| z42n_1p1v_it.ibs  *  IBIS 5.0 Model
| 16Gb Mobile LPDDR4 SDRAM - Die Revision E
| This Model is valid for Automotive A2 Temperature Range  -40C<=Ta<=105C
| Part Number   VDD2/VDDQ   Architecture  Package
| SCE11U64324EF   1.10/1.10   1024M x 32   TFBGA (200b,DDP,10x14.5x1.1)
[IBIS Ver]  5.0
[File Name] z42n_0p6v_it.ibs
[Date]   03/31/2025
[File Rev]  2.3
[Source]   Unisemicon, Inc.
[Notes]
   Date   Revision   Contents
   March 31, 2025   1.00   Initial release
[Disclaimer]THESE IBIS MODELS ARE PROVIDED "AS IS" WITH NO WARRANTY AND Unisemicon IS NOT RESPONSIBLE FOR ANY PROBLEMS
   THIS MODEL MAY CAUSE TO THE CUSTOMERS. THESE MODELS ARE SUBJECT TO CHANGE WITHOUT ANY NOTICE.
[Copyright]   Copyright 2025 UniIC, Inc. All rights reserved.
| C_COMP Data:
|   typ   min   max
| DQ   0.834pF   0.784pF   0.884pF
| DQS   0.849pF   0.799pF   0.899pF
| CA_INPUT   0.679pF   0.629pF   0.729pF
| CS_INPUT   0.655pF   0.605pF   0.705pF
| CLK_INPUT   0.656pF   0.606pF   0.706pF
| CKE_INPUT   0.683pF   0.633pF   0.733pF
| ODTCA_INPUT   0.625pF   0.575pF   0.675pF
|COMPONENT:[ SCE11U64324EF ]
[Component]   SCE11U64324EF
[Package Model]  Z42N_200B_SDP_LB2
[Manufacturer]   xxx Technology, Inc.
[Package]
|   typ   min   max
R_pkg   603.13m   431.42m   899.94m
L_pkg   1.668nH   1.132nH   2.472nH
C_pkg   0.609pF   0.467pF   0.865pF
[Pin] signal_name  model_name   R_pin   L_pin   C_pin   | TD_pin(ps)   Z_pin
A1   DNU   NC
A2   DNU   NC
A3   VSS   GND
A4   VDD2   POWER
A5   ZQ   NC
A8   NC   NC
A9   VDD2   POWER
A10   VSS   GND
A11   DNU   NC
A12   DNU   NC
B1   DNU   NC
B2   DQ0   DQ   579.30m   1.530nH   0.601pF   |  30.324   50.455
B3   VDDQ   POWER
B4   DQ7   DQ   521.60m   1.376nH   0.535pF   |  27.132   50.715
B5   VDDQ   POWER
B8   VDDQ   POWER
B9   DQ15   DQ   521.58m   1.381nH   0.535pF   |  27.182   50.807
B10   VDDQ   POWER
B11   DQ8   DQ   582.09m   1.533nH   0.605pF   |  30.454   50.338
B12   DNU   NC
C1   VSS   GND
C2   DQ1   DQ   508.10m   1.311nH   0.554pF   |  26.950   48.646
C3   DMI0   DQ   443.13m   1.164nH   0.502pF   |  24.173   48.153
C4   DQ6   DQ   454.87m   1.195nH   0.489pF   |  24.173   49.434
C5   VSS   GND
C8   VSS   GND
C9   DQ14   DQ   452.17m   1.190nH   0.488pF   |  24.098   49.381
C10   DMI1   DQ   446.55m   1.178nH   0.502pF   |  24.318   48.442
C11   DQ9   DQ   508.55m   1.324nH   0.556pF   |  27.132   48.799
C12   VSS   GND
D1   VDDQ   POWER
D2   VSS   GND
D3   DQS0_t   DQS   651.43m   1.905nH   0.628pF   |  34.588   55.077
D4   VSS   GND
D5   VDDQ   POWER
D8   VDDQ   POWER
D9   VSS   GND
D10   DQS1_t   DQS   651.42m   1.914nH   0.629pF   |  34.697   55.163
D11   VSS   GND
D12   VDDQ   POWER
E1   VSS   GND
E2   DQ2   DQ   500.68m   1.348nH   0.529pF   |  26.704   50.480
E3   DQS0_c   DQS   643.34m   1.890nH   0.601pF   |  33.703   56.078
E4   DQ5   DQ   431.42m   1.168nH   0.481pF   |  23.702   49.278
E5   VSS   GND
E8   VSS   GND
E9   DQ13   DQ   431.43m   1.169nH   0.486pF   |  23.836   49.044
E10   DQS1_c   DQS   643.50m   1.890nH   0.601pF   |  33.703   56.078
E11   DQ10   DQ   500.70m   1.345nH   0.529pF   |  26.674   50.424
E12   VSS   GND
F1   VDD1   POWER
F2   DQ3   DQ   550.84m   1.447nH   0.577pF   |  28.895   50.078
F3   VDDQ   POWER
F4   DQ4   DQ   438.89m   1.132nH   0.467pF   |  22.992   49.234
F5   VDD2   POWER
F8   VDD2   POWER
F9   DQ12   DQ   438.92m   1.132nH   0.472pF   |  23.115   48.972
F10   VDDQ   POWER
F11   DQ11   DQ   550.98m   1.456nH   0.577pF   |  28.985   50.233
F12   VDD1   POWER
G1   VSS   GND
G2   ODT_CA   ODTCA_INPUT   748.07m   2.139nH   0.691pF   |  38.445   55.637
G3   VSS   GND
G4   VDD1   POWER
G5   VSS   GND
G8   VSS   GND
G9   VDD1   POWER
G10   VSS   GND
G11   NC   NC
G12   VSS   GND
H1   VDD2   POWER
H2   CA0   CA_INPUT   811.90m   2.235nH   0.759pF   |  41.187   54.265
H3   NC   NC
H4   CS   CS_INPUT   646.92m   1.910nH   0.647pF   |  35.154   54.333
H5   VDD2   POWER
H8   VDD2   POWER
H9   CA2   CA_INPUT   693.42m   1.911nH   0.688pF   |  36.260   52.703
H10   CA3   CA_INPUT   772.58m   2.175nH   0.746pF   |  40.281   53.996
H11   CA4   CA_INPUT   845.75m   2.405nH   0.802pF   |  43.918   54.761
H12   VDD2   POWER
J1   VSS   GND
J2   CA1   CA_INPUT   872.08m   2.359nH   0.844pF   |  44.621   52.868
J3   VSS   GND
J4   CKE   CKE_INPUT   683.83m   2.042nH   0.679pF   |  37.236   54.839
J5   NC   NC
J8   CK_t   CLK_INPUT   739.69m   2.222nH   0.719pF   |  39.970   55.591
J9   CK_c   CLK_INPUT   737.69m   2.200nH   0.716pF   |  39.689   55.431
J10   VSS   GND
J11   CA5   CA_INPUT   899.94m   2.472nH   0.865pF   |  46.242   53.458
J12   VSS   GND
K1   VDD2   POWER
K2   VSS   GND
K3   VDD2   POWER
K4   VSS   GND
K5   NC   NC
K8   NC   NC
K9   VSS   GND
K10   VDD2   POWER
K11   VSS   GND
K12   VDD2   POWER
N1   VDD2   POWER
N2   VSS   GND
N3   VDD2   POWER
N4   VSS   GND
N5   NC   NC
N8   NC   NC
N9   VSS   GND
N10   VDD2   POWER
N11   VSS   GND
N12   VDD2   POWER
P1   VSS   GND
P2   NC   NC
P3   VSS   GND
P4   NC   NC
P5   NC   NC
P8   NC   NC
P9   NC   NC
P10   VSS   GND
P11   NC   NC
P12   VSS   GND
R1   VDD2   POWER
R2   NC   NC
R3   NC   NC
R4   NC   NC
R5   VDD2   POWER
R8   VDD2   POWER
R9   NC   NC
R10   NC   NC
R11   NC   NC
R12   VDD2   POWER
T1   VSS   GND
T2   NC   NC
T3   VSS   GND
T4   VDD1   POWER
T5   VSS   GND
T8   VSS   GND
T9   VDD1   POWER
T10   VSS   GND
T11   RESET_n   NC
T12   VSS   GND
U1   VDD1   POWER
U2   NC   NC
U3   VDDQ   POWER
U4   NC   NC
U5   VDD2   POWER
U8   VDD2   POWER
U9   NC   NC
U10   VDDQ   POWER
U11   NC   NC
U12   VDD1   POWER
V1   VSS   GND
V2   NC   NC
V3   NC   NC
V4   NC   NC
V5   VSS   GND
V8   VSS   GND
V9   NC   NC
V10   NC   NC
V11   NC   NC
V12   VSS   GND
W1   VDDQ   POWER
W2   VSS   GND
W3   NC   NC
W4   VSS   GND
W5   VDDQ   POWER
W8   VDDQ   POWER
W9   VSS   GND
W10   NC   NC
W11   VSS   GND
W12   VDDQ   POWER
Y1   VSS   GND
Y2   NC   NC
Y3   NC   NC
Y4   NC   NC
Y5   VSS   GND
Y8   VSS   GND
Y9   NC   NC
Y10   NC   NC
Y11   NC   NC
Y12   VSS   GND
AA1   DNU   NC
AA2   NC   NC
AA3   VDDQ   POWER
AA4   NC   NC
AA5   VDDQ   POWER
AA8   VDDQ   POWER
AA9   NC   NC
AA10  VDDQ   POWER
AA11  NC   NC
AA12  DNU   NC
AB1   DNU   NC
AB2   DNU   NC
AB3   VSS   GND
AB4   VDD2   POWER
AB5   VSS   GND
AB8   VSS   GND
AB9   VDD2   POWER
AB10  VSS   GND
AB11  DNU   NC
AB12  DNU   NC
|*****  PIN MAPPING  *******************************************************
[Pin Mapping] pulldown_ref pullup_ref gnd_clamp_ref power_clamp_ref ext_ref
A1   NC   NC
A2   NC   NC
A3   VSS   NC
A4   NC   VDD2
A5   NC   NC
A8   NC   NC
A9   NC   VDD2
A10   VSS   NC
A11   NC   NC
A12   NC   NC
B1   NC   NC
B2   VSS   VDDQ   VSS   VDDQ
B3   NC   VDDQ
B4   VSS   VDDQ   VSS   VDDQ
B5   NC   VDDQ
B8   NC   VDDQ
B9   VSS   VDDQ   VSS   VDDQ
B10   NC   VDDQ
B11   VSS   VDDQ   VSS   VDDQ
B12   NC   NC
C1   VSS   NC
C2   VSS   VDDQ   VSS   VDDQ
C3   VSS   VDDQ   VSS   VDDQ
C4   VSS   VDDQ   VSS   VDDQ
C5   VSS   NC
C8   VSS   NC
C9   VSS   VDDQ   VSS   VDDQ
C10   VSS   VDDQ   VSS   VDDQ
C11   VSS   VDDQ   VSS   VDDQ
C12   VSS   NC
D1   NC   VDDQ
D2   VSS   NC
D3   VSS   VDDQ   VSS   VDDQ
D4   VSS   NC
D5   NC   VDDQ
D8   NC   VDDQ
D9   VSS   NC
D10   VSS   VDDQ   VSS   VDDQ
D11   VSS   NC
D12   NC   VDDQ
E1   VSS   NC
E2   VSS   VDDQ   VSS   VDDQ
E3   VSS   VDDQ   VSS   VDDQ
E4   VSS   VDDQ   VSS   VDDQ
E5   VSS   NC
E8   VSS   NC
E9   VSS   VDDQ   VSS   VDDQ
E10   VSS   VDDQ   VSS   VDDQ
E11   VSS   VDDQ   VSS   VDDQ
E12   VSS   NC
F1   NC   VDD1
F2   VSS   VDDQ   VSS   VDDQ
F3   NC   VDDQ
F4   VSS   VDDQ   VSS   VDDQ
F5   NC   VDD2
F8   NC   VDD2
F9   VSS   VDDQ   VSS   VDDQ
F10   NC   VDDQ
F11   VSS   VDDQ   VSS   VDDQ
F12   NC   VDD1
G1   VSS   NC
G2   NC   NC   VSS   VDD2
G3   VSS   NC
G4   NC   VDD1
G5   VSS   NC
G8   VSS   NC
G9   NC   VDD1
G10   VSS   NC
G11   NC   NC
G12   VSS   NC
H1   NC   VDD2
H2   NC   NC   VSS   VDD2
H3   NC   NC
H4   NC   NC   VSS   VDD2
H5   NC   VDD2
H8   NC   VDD2
H9   NC   NC   VSS   VDD2
H10   NC   NC   VSS   VDD2
H11   NC   NC   VSS   VDD2
H12   NC   VDD2
J1   VSS   NC
J2   NC   NC   VSS   VDD2
J3   VSS   NC
J4   NC   NC   VSS   VDD2
J5   NC   NC
J8   NC   NC   VSS   VDD2
J9   NC   NC   VSS   VDD2
J10   VSS   NC
J11   NC   NC   VSS   VDD2
J12   VSS   NC
K1   NC   VDD2
K2   VSS   NC
K3   NC   VDD2
K4   VSS   NC
K5   NC   NC
K8   NC   NC
K9   VSS   NC
K10   NC   VDD2
K11   VSS   NC
K12   NC   VDD2
N1   NC   VDD2
N2   VSS   NC
N3   NC   VDD2
N4   VSS   NC
N5   NC   NC
N8   NC   NC
N9   VSS   NC
N10   NC   VDD2
N11   VSS   NC
N12   NC   VDD2
P1   VSS   NC
P2   NC   NC
P3   VSS   NC
P4   NC   NC
P5   NC   NC
P8   NC   NC
P9   NC   NC
P10   VSS   NC
P11   NC   NC
P12   VSS   NC
R1   NC   VDD2
R2   NC   NC
R3   NC   NC
R4   NC   NC
R5   NC   VDD2
R8   NC   VDD2
R9   NC   NC
R10   NC   NC
R11   NC   NC
R12   NC   VDD2
T1   VSS   NC
T2   NC   NC
T3   VSS   NC
T4   NC   VDD1
T5   VSS   NC
T8   VSS   NC
T9   NC   VDD1
T10   VSS   NC
T11   NC   NC
T12   VSS   NC
U1   NC   VDD1
U2   NC   NC
U3   NC   VDDQ
U4   NC   NC
U5   NC   VDD2
U8   NC   VDD2
U9   NC   NC
U10   NC   VDDQ
U11   NC   NC
U12   NC   VDD1
V1   VSS   NC
V2   NC   NC
V3   NC   NC
V4   NC   NC
V5   VSS   NC
V8   VSS   NC
V9   NC   NC
V10   NC   NC
V11   NC   NC
V12   VSS   NC
W1   NC   VDDQ
W2   VSS   NC
W3   NC   NC
W4   VSS   NC
W5   NC   VDDQ
W8   NC   VDDQ
W9   VSS   NC
W10   NC   NC
W11   VSS   NC
W12   NC   VDDQ
Y1   VSS   NC
Y2   NC   NC
Y3   NC   NC
Y4   NC   NC
Y5   VSS   NC
Y8   VSS   NC
Y9   NC   NC
Y10   NC   NC
Y11   NC   NC
Y12   VSS   NC
AA1   NC   NC
AA2   NC   NC
AA3   NC   VDDQ
AA4   NC   NC
AA5   NC   VDDQ
AA8   NC   VDDQ
AA9   NC   NC
AA10   NC   VDDQ
AA11   NC   NC
AA12   NC   NC
AB1   NC   NC
AB2   NC   NC
AB3   VSS   NC
AB4   NC   VDD2
AB5   VSS   NC
AB8   VSS   NC
AB9   NC   VDD2
AB10   VSS   NC
AB11   NC   NC
AB12   NC   NC
|*****  DIFF PIN  **********************************************************
[Diff Pin]  inv_pin  vdiff   tdelay_typ   tdelay_min   tdelay_max
D3   E3   0.120V   0.000s   NA   NA
D10   E10   0.120V   0.000s   NA   NA
J8   J9   0.145V   0.000s   NA   NA
|END COMPONENT *************************************************************
|COMPONENT:[ MT53E1G32D2FW ]
[Component]   MT53E1G32D2FW
[Package Model]  Z42N_200B_DDP_LB2
[Manufacturer]   xxx Technology, Inc.
[Package]
|   typ   min   max
R_pkg   1781m   683m   3340m
L_pkg   3.313nH   1.222nH   6.06nH
C_pkg   1.15pF   0.604pF   2.03pF
[Pin] signal_name  model_name   R_pin   L_pin   C_pin
A1   DNU   NC
A2   DNU   NC
A3   VSS   GND
A4   VDD2   POWER
A5   ZQ0   NC
A8   ZQ1   NC
A9   VDD2   POWER
A10   VSS   GND
A11   DNU   NC
A12   DNU   NC
B1   DNU   NC
B2   DQ0_A   DQ   892.22m   1.783nH   0.667pF
B3   VDDQ   POWER
B4   DQ7_A   DQ   942.05m   1.831nH   0.712pF
B5   VDDQ   POWER
B8   VDDQ   POWER
B9   DQ15_A   DQ   905.71m   1.724nH   0.652pF
B10   VDDQ   POWER
B11   DQ8_A   DQ   951.2m   1.847nH   0.708pF
B12   DNU   NC
C1   VSS   GND
C2   DQ1_A   DQ   869.4m   1.675nH   0.663pF
C3   DMI0_A   DQ   802.2m   1.539nH   0.644pF
C4   DQ6_A   DQ   695.07m   1.386nH   0.604pF
C5   VSS   GND
C8   VSS   GND
C9   DQ14_A   DQ   809.8m   1.568nH   0.657pF
C10   DMI1_A   DQ   843.49m   1.585nH   0.669pF
C11   DQ9_A   DQ   862.4m   1.663nH   0.667pF
C12   VSS   GND
D1   VDDQ   POWER
D2   VSS   GND
D3   DQS0_t_A   DQS   872.77m   1.603nH   0.663pF
D4   VSS   GND
D5   VDDQ   POWER
D8   VDDQ   POWER
D9   VSS   GND
D10   DQS1_t_A   DQS   906.95m   1.659nH   0.687pF
D11   VSS   GND
D12   VDDQ   POWER
E1   VSS   GND
E2   DQ2_A   DQ   766.79m   1.41nH   0.641pF
E3   DQS0_c_A   DQS   892.7m   1.616nH   0.682pF
E4   DQ5_A   DQ   683.1m   1.243nH   0.617pF
E5   VSS   GND
E8   VSS   GND
E9   DQ13_A   DQ   751.68m   1.328nH   0.636pF
E10   DQS1_c_A   DQS   932m   1.697nH   0.709pF
E11   DQ10_A   DQ   805.68m   1.499nH   0.658pF
E12   VSS   GND
F1   VDD1   POWER
F2   DQ3_A   DQ   815.2m   1.487nH   0.658pF
F3   VDDQ   POWER
F4   DQ4_A   DQ   684.7m   1.222nH   0.624pF
F5   VDD2   POWER
F8   VDD2   POWER
F9   DQ12_A   DQ   754m   1.333nH   0.665pF
F10   VDDQ   POWER
F11   DQ11_A   DQ   816.75m   1.527nH   0.656pF
F12   VDD1   POWER
G1   VSS   GND
G2   ODT_CA_A   ODTCA_INPUT   3223m   5.38nH   0.839pF
G3   VSS   GND
G4   VDD1   POWER
G5   VSS   GND
G8   VSS   GND
G9   VDD1   POWER
G10   VSS   GND
G11   NC   NC
G12   VSS   GND
H1   VDD2   POWER
H2   CA0_A   CA_INPUT   1381m   2.44nH   0.952pF
H3   NC   NC
H4   CS0_A   CS_INPUT
H5   VDD2   POWER
H8   VDD2   POWER
H9   CA2_A   CA_INPUT   1146m   2.055nH   0.856pF
H10   CA3_A   CA_INPUT   1283m   2.28nH   0.92pF
H11   CA4_A   CA_INPUT   1456m   2.59nH   1.005pF
H12   VDD2   POWER
J1   VSS   GND
J2   CA1_A   CA_INPUT   1531m   2.64nH   1.061pF
J3   VSS   GND
J4   CKE0_A   CKE_INPUT
J5   NC   NC
J8   CK_t_A   CLK_INPUT   1327m   2.423nH   0.917pF
J9   CK_c_A   CLK_INPUT   1352m   2.46nH   0.936pF
J10   VSS   GND
J11   CA5_A   CA_INPUT   1682m   2.901nH   1.08pF
J12   VSS   GND
K1   VDD2   POWER
K2   VSS   GND
K3   VDD2   POWER
K4   VSS   GND
K5   NC   NC
K8   NC   NC
K9   VSS   GND
K10   VDD2   POWER
K11   VSS   GND
K12   VDD2   POWER
N1   VDD2   POWER
N2   VSS   GND
N3   VDD2   POWER
N4   VSS   GND
N5   NC   NC
N8   NC   NC
N9   VSS   GND
N10   VDD2   POWER
N11   VSS   GND
N12   VDD2   POWER
P1   VSS   GND
P2   CA1_B   CA_INPUT   2001m   3.59nH   1.24pF
P3   VSS   GND
P4   CKE0_B   CKE_INPUT
P5   NC   NC
P8   CK_t_B   CLK_INPUT   1908m   3.371nH   1.215pF
P9   CK_c_B   CLK_INPUT   1352m   2.464nH   0.936pF
P10   VSS   GND
P11   CA5_B   CA_INPUT   1935m   3.552nH   1.192pF
P12   VSS   GND
R1   VDD2   POWER
R2   CA0_B   CA_INPUT   2110m   3.79nH   1.283pF
R3   NC   NC
R4   CS0_B   CS_INPUT
R5   VDD2   POWER
R8   VDD2   POWER
R9   CA2_B   CA_INPUT   1965m   3.398nH   1.229pF
R10   CA3_B   CA_INPUT   2061m   3.706nH   1.26pF
R11   CA4_B   CA_INPUT   1859m   3.388nH   1.151pF
R12   VDD2   POWER
T1   VSS   GND
T2   ODT_CA_B   ODTCA_INPUT   1974m   3.548nH   1.128pF
T3   VSS   GND
T4   VDD1   POWER
T5   VSS   GND
T8   VSS   GND
T9   VDD1   POWER
T10   VSS   GND
T11   RESET_n   NC
T12   VSS   GND
U1   VDD1   POWER
U2   DQ3_B   DQ   2687m   4.766nH   1.558pF
U3   VDDQ   POWER
U4   DQ4_B   DQ   2425m   4.233nH   1.469pF
U5   VDD2   POWER
U8   VDD2   POWER
U9   DQ12_B   DQ   3116m   5.207nH   1.812pF
U10   VDDQ   POWER
U11   DQ11_B   DQ   3179m   5.321nH   1.828pF
U12   VDD1   POWER
V1   VSS   GND
V2   DQ2_B   DQ   2588m   4.551nH   1.513pF
V3   DQS0_c_B   DQS   2438m   4.346nH   1.466pF
V4   DQ5_B   DQ   2290m   4.012nH   1.391pF
V5   VSS   GND
V8   VSS   GND
V9   DQ13_B   DQ   3013m   5.038nH   1.759pF
V10   DQS1_c_B   DQS   3073m   5.198nH   1.833pF
V11   DQ10_B   DQ   3240m   5.404nH   1.898pF
V12   VSS   GND
W1   VDDQ   POWER
W2   VSS   GND
W3   DQS0_t_B   DQS   2438m   4.346nH   1.466pF
W4   VSS   GND
W5   VDDQ   POWER
W8   VDDQ   POWER
W9   VSS   GND
W10   DQS1_t_B   DQS   3167m   5.386nH   1.871pF
W11   VSS   GND
W12   VDDQ   POWER
Y1   VSS   GND
Y2   DQ1_B   DQ   2484m   4.410nH   1.467pF
Y3   DMI0_B   DQ   2282m   4.056nH   1.378pF
Y4   DQ6_B   DQ   2149m   3.822nH   1.313pF
Y5   VSS   GND
Y8   VSS   GND
Y9   DQ14_B   DQ   3051m   5.183nH   1.804pF
Y10   DMI1_B   DQ   3195m   5.155nH   1.899pF
Y11   DQ9_B   DQ   3347m   5.68nH   1.932pF
Y12   VSS   GND
AA1   DNU   NC
AA2   DQ0_B   DQ   2472m   4.484nH   1.453pF
AA3   VDDQ   POWER
AA4   DQ7_B   DQ   2196m   4.004nH   1.284pF
AA5   VDDQ   POWER
AA8   VDDQ   POWER
AA9   DQ15_B   DQ   3046m   5.081nH   1.82pF
AA10  VDDQ   POWER
AA11  DQ8_B   DQ   3565m   6.06nH   2.037pF
AA12  DNU   NC
AB1   DNU   NC
AB2   DNU   NC
AB3   VSS   GND
AB4   VDD2   POWER
AB5   VSS   GND
AB8   VSS   GND
AB9   VDD2   POWER
AB10  VSS   GND
AB11  DNU   NC
AB12  DNU   NC
|*****  PIN MAPPING  *******************************************************
[Pin Mapping] pulldown_ref pullup_ref gnd_clamp_ref power_clamp_ref ext_ref
A1   NC   NC
A2   NC   NC
A3   VSS   NC
A4   NC   VDD2
A5   NC   NC
A8   NC   NC
A9   NC   VDD2
A10   VSS   NC
A11   NC   NC
A12   NC   NC
B1   NC   NC
B2   VSS   VDDQ   VSS   VDDQ
B3   NC   VDDQ
B4   VSS   VDDQ   VSS   VDDQ
B5   NC   VDDQ
B8   NC   VDDQ
B9   VSS   VDDQ   VSS   VDDQ
B10   NC   VDDQ
B11   VSS   VDDQ   VSS   VDDQ
B12   NC   NC
C1   VSS   NC
C2   VSS   VDDQ   VSS   VDDQ
C3   VSS   VDDQ   VSS   VDDQ
C4   VSS   VDDQ   VSS   VDDQ
C5   VSS   NC
C8   VSS   NC
C9   VSS   VDDQ   VSS   VDDQ
C10   VSS   VDDQ   VSS   VDDQ
C11   VSS   VDDQ   VSS   VDDQ
C12   VSS   NC
D1   NC   VDDQ
D2   VSS   NC
D3   VSS   VDDQ   VSS   VDDQ
D4   VSS   NC
D5   NC   VDDQ
D8   NC   VDDQ
D9   VSS   NC
D10   VSS   VDDQ   VSS   VDDQ
D11   VSS   NC
D12   NC   VDDQ
E1   VSS   NC
E2   VSS   VDDQ   VSS   VDDQ
E3   VSS   VDDQ   VSS   VDDQ
E4   VSS   VDDQ   VSS   VDDQ
E5   VSS   NC
E8   VSS   NC
E9   VSS   VDDQ   VSS   VDDQ
E10   VSS   VDDQ   VSS   VDDQ
E11   VSS   VDDQ   VSS   VDDQ
E12   VSS   NC
F1   NC   VDD1
F2   VSS   VDDQ   VSS   VDDQ
F3   NC   VDDQ
F4   VSS   VDDQ   VSS   VDDQ
F5   NC   VDD2
F8   NC   VDD2
F9   VSS   VDDQ   VSS   VDDQ
F10   NC   VDDQ
F11   VSS   VDDQ   VSS   VDDQ
F12   NC   VDD1
G1   VSS   NC
G2   NC   NC   VSS   VDD2
G3   VSS   NC
G4   NC   VDD1
G5   VSS   NC
G8   VSS   NC
G9   NC   VDD1
G10   VSS   NC
G11   NC   NC
G12   VSS   NC
H1   NC   VDD2
H2   NC   NC   VSS   VDD2
H3   NC   NC
H4   NC   NC   VSS   VDD2
H5   NC   VDD2
H8   NC   VDD2
H9   NC   NC   VSS   VDD2
H10   NC   NC   VSS   VDD2
H11   NC   NC   VSS   VDD2
H12   NC   VDD2
J1   VSS   NC
J2   NC   NC   VSS   VDD2
J3   VSS   NC
J4   NC   NC   VSS   VDD2
J5   NC   NC
J8   NC   NC   VSS   VDD2
J9   NC   NC   VSS   VDD2
J10   VSS   NC
J11   NC   NC   VSS   VDD2
J12   VSS   NC
K1   NC   VDD2
K2   VSS   NC
K3   NC   VDD2
K4   VSS   NC
K5   NC   NC
K8   NC   NC
K9   VSS   NC
K10   NC   VDD2
K11   VSS   NC
K12   NC   VDD2
N1   NC   VDD2
N2   VSS   NC
N3   NC   VDD2
N4   VSS   NC
N5   NC   NC
N8   NC   NC
N9   VSS   NC
N10   NC   VDD2
N11   VSS   NC
N12   NC   VDD2
P1   VSS   NC
P2   NC   NC   VSS   VDD2
P3   VSS   NC
P4   NC   NC   VSS   VDD2
P5   NC   NC
P8   NC   NC   VSS   VDD2
P9   NC   NC   VSS   VDD2
P10   VSS   NC
P11   NC   NC   VSS   VDD2
P12   VSS   NC
R1   NC   VDD2
R2   NC   NC   VSS   VDD2
R3   NC   NC
R4   NC   NC   VSS   VDD2
R5   NC   VDD2
R8   NC   VDD2
R9   NC   NC   VSS   VDD2
R10   NC   NC   VSS   VDD2
R11   NC   NC   VSS   VDD2
R12   NC   VDD2
T1   VSS   NC
T2   NC   NC   VSS   VDD2
T3   VSS   NC
T4   NC   VDD1
T5   VSS   NC
T8   VSS   NC
T9   NC   VDD1
T10   VSS   NC
T11   NC   NC
T12   VSS   NC
U1   NC   VDD1
U2   VSS   VDDQ   VSS   VDDQ
U3   NC   VDDQ
U4   VSS   VDDQ   VSS   VDDQ
U5   NC   VDD2
U8   NC   VDD2
U9   VSS   VDDQ   VSS   VDDQ
U10   NC   VDDQ
U11   VSS   VDDQ   VSS   VDDQ
U12   NC   VDD1
V1   VSS   NC
V2   VSS   VDDQ   VSS   VDDQ
V3   VSS   VDDQ   VSS   VDDQ
V4   VSS   VDDQ   VSS   VDDQ
V5   VSS   NC
V8   VSS   NC
V9   VSS   VDDQ   VSS   VDDQ
V10   VSS   VDDQ   VSS   VDDQ
V11   VSS   VDDQ   VSS   VDDQ
V12   VSS   NC
W1   NC   VDDQ
W2   VSS   NC
W3   VSS   VDDQ   VSS   VDDQ
W4   VSS   NC
W5   NC   VDDQ
W8   NC   VDDQ
W9   VSS   NC
W10   VSS   VDDQ   VSS   VDDQ
W11   VSS   NC
W12   NC   VDDQ
Y1   VSS   NC
Y2   VSS   VDDQ   VSS   VDDQ
Y3   VSS   VDDQ   VSS   VDDQ
Y4   VSS   VDDQ   VSS   VDDQ
Y5   VSS   NC
Y8   VSS   NC
Y9   VSS   VDDQ   VSS   VDDQ
Y10   VSS   VDDQ   VSS   VDDQ
Y11   VSS   VDDQ   VSS   VDDQ
Y12   VSS   NC
AA1   NC   NC
AA2   VSS   VDDQ   VSS   VDDQ
AA3   NC   VDDQ
AA4   VSS   VDDQ   VSS   VDDQ
AA5   NC   VDDQ
AA8   NC   VDDQ
AA9   VSS   VDDQ   VSS   VDDQ
AA10   NC   VDDQ
AA11   VSS   VDDQ   VSS   VDDQ
AA12   NC   NC
AB1   NC   NC
AB2   NC   NC
AB3   VSS   NC
AB4   NC   VDD2
AB5   VSS   NC
AB8   VSS   NC
AB9   NC   VDD2
AB10   VSS   NC
AB11   NC   NC
AB12   NC   NC
|*****  DIFF PIN  **********************************************************
[Diff Pin]  inv_pin  vdiff   tdelay_typ   tdelay_min   tdelay_max
D3   E3   0.120V   0.000s   NA   NA
W3   V3   0.120V   0.000s   NA   NA
D10   E10   0.120V   0.000s   NA   NA
W10   V10   0.120V   0.000s   NA   NA
J8   J9   0.145V   0.000s   NA   NA
P8   P9   0.145V   0.000s   NA   NA
|END COMPONENT *************************************************************
|COMPONENT:[ MT53E1G64D4NZ ]
[Component]   MT53E1G64D4NZ
[Package Model]  Z42N_376B_PKG
[Manufacturer]   xxx Technology, Inc.
[Package]
|   typ   min   max
R_pkg   548.13m   401.67m   805.14m
L_pkg   1.106nH   0.844nH   1.656nH
C_pkg   0.528pF   0.405pF   0.790pF
[Pin] signal_name  model_name   R_pin   L_pin   C_pin   | TD_pin(ps)   Z_pin
A1   NC   NC
A2   VDD2   POWER
A3   DQ3_A   DQ   582.00m   1.144nH   0.562pF   |  25.356   45.117
A4   VSS   GND
A5   DQ5_A   DQ   563.12m   1.109nH   0.546pF   |  24.607   45.068
A6   ODT_ca_A   ODTCA_INPUT   588.02m   1.213nH   0.556pF   |  25.970   46.708
A7   CA0_A   CA_INPUT   586.92m   1.232nH   0.555pF   |  26.149   47.115
A10   CA2_A   CA_INPUT   551.96m   1.159nH   0.529pF   |  24.761   46.807
A11   VSS   GND
A12   VSS   GND
A13   DQ13_A   DQ   569.49m   1.112nH   0.553pF   |  24.798   44.843
A14   VDD2   POWER
A15   VDD1   POWER
A16   DQ10_A   DQ   591.32m   1.187nH   0.567pF   |  25.943   45.755
A17   ZQ1_A   NC
A18   ZQ1_D   NC
A19   DQ10_C   DQ   594.16m   1.186nH   0.569pF   |  25.978   45.655
A20   VDD1   POWER
A21   VDD2   POWER
A22   DQ13_C   DQ   570.38m   1.112nH   0.554pF   |  24.820   44.802
A23   VSS   GND
A24   VSS   GND
A25   CA2_C   CA_INPUT   559.40m   1.184nH   0.580pF   |  26.205   45.182
A28   CA0_C   CA_INPUT   558.35m   1.198nH   0.587pF   |  26.518   45.176
A29   ODT_ca_C   ODTCA_INPUT   788.52m   1.615nH   0.774pF   |  35.355   45.679
A30   DQ5_C   DQ   561.90m   1.108nH   0.546pF   |  24.596   45.048
A31   VSS   GND
A32   DQ3_C   DQ   583.56m   1.146nH   0.562pF   |  25.378   45.157
A33   VDD2   POWER
A34   NC   NC
B1   VSS   GND
B2   DQ2_A   DQ   544.67m   1.066nH   0.507pF   |  23.248   45.854
B3   VDDQ   POWER
B4   DMI0_A   DQ   522.70m   1.021nH   0.487pF   |  22.299   45.788
B5   VDDQ   POWER
B6   DQ7_A   DQ   505.86m   0.986nH   0.473pF   |  21.596   45.657
B7   VDD2   POWER
B8   CS0_A   CS_INPUT   484.51m   1.020nH   0.451pF   |  21.448   47.557
B9   CKE0_A   CKE_INPUT   514.27m   1.070nH   0.471pF   |  22.449   47.663
B10   VDD2   POWER
B11   CA4_A   CA_INPUT   493.44m   1.018nH   0.459pF   |  21.616   47.094
B12   DQ15_A   DQ   498.18m   0.972nH   0.468pF   |  21.328   45.573
B13   VDDQ   POWER
B14   DMI1_A   DQ   515.91m   1.014nH   0.481pF   |  22.085   45.914
B15   DQ11_A   DQ   520.48m   1.020nH   0.488pF   |  22.311   45.718
B16   VSS   GND
B17   ZQ0_A   NC
B18   ZQ0_D   NC
B19   VSS   GND
B20   DQ11_C   DQ   523.13m   1.021nH   0.489pF   |  22.344   45.694
B21   DMI1_C   DQ   516.78m   1.021nH   0.481pF   |  22.161   46.072
B22   VDDQ   POWER
B23   DQ15_C   DQ   499.65m   0.967nH   0.470pF   |  21.319   45.359
B24   CA4_C   CA_INPUT   474.96m   0.995nH   0.501pF   |  22.327   44.565
B25   VDD2   POWER
B26   CKE0_C   CKE_INPUT   502.58m   1.052nH   0.505pF   |  23.049   45.642
B27   CS0_C   CS_INPUT   589.85m   1.235nH   0.536pF   |  25.729   48.001
B28   VDD2   POWER
B29   DQ7_C   DQ   503.56m   0.982nH   0.471pF   |  21.506   45.661
B30   VDDQ   POWER
B31   DMI0_C   DQ   523.29m   1.023nH   0.487pF   |  22.320   45.832
B32   VDDQ   POWER
B33   DQ2_C   DQ   545.83m   1.069nH   0.508pF   |  23.303   45.873
B34   VSS   GND
C1   DQ0_A   DQ   551.19m   1.096nH   0.507pF   |  23.573   46.494
C2   VDDQ   POWER
C3   VSS   GND
C4   VSS   GND
C5   DQ4_A   DQ   451.07m   0.876nH   0.429pF   |  19.386   45.188
C6   VDDQ   POWER
C7   CA1_A   CA_INPUT   439.67m   0.924nH   0.417pF   |  19.629   47.073
C8   VDD2   POWER
C9   VSS   GND
C10   CA3_A   CA_INPUT   429.31m   0.896nH   0.405pF   |  19.049   47.036
C11   VSS   GND
C12   VDDQ   POWER
C13   DQ12_A   DQ   432.12m   0.844nH   0.419pF   |  18.805   44.881
C14   VSS   GND
C15   VDDQ   POWER
C16   DQ9_A   DQ   482.64m   0.945nH   0.457pF   |  20.781   45.473
C17   RESET_n   NC
C18   NC   NC
C19   DQ9_C   DQ   485.66m   0.942nH   0.458pF   |  20.771   45.352
C20   VDDQ   POWER
C21   VSS   GND
C22   DQ12_C   DQ   434.93m   0.845nH   0.420pF   |  18.839   44.854
C23   VDDQ   POWER
C24   VSS   GND
C25   CA3_C   CA_INPUT   401.67m   0.866nH   0.434pF   |  19.387   44.670
C26   VSS   GND
C27   VDD2   POWER
C28   CA1_C   CA_INPUT   420.28m   0.891nH   0.440pF   |  19.800   45.000
C29   VDDQ   POWER
C30   DQ4_C   DQ   450.94m   0.876nH   0.430pF   |  19.408   45.135
C31   VSS   GND
C32   VSS   GND
C33   VDDQ   POWER
C34   DQ0_C   DQ   550.68m   1.095nH   0.505pF   |  23.515   46.565
D1   VDD1   POWER
D2   DQ1_A   DQ   482.26m   0.945nH   0.455pF   |  20.736   45.573
D3   DQS0_t_A   DQS   619.19m   1.246nH   0.595pF   |  27.228   45.762
D4   DQS0_c_A   DQS   617.64m   1.252nH   0.592pF   |  27.225   45.988
D5   VSS   GND
D6   DQ6_A   DQ   561.92m   1.086nH   0.558pF   |  24.617   44.116
D7   VSS   GND
D8   CK_t_A   CLK_INPUT   587.34m   1.196nH   0.562pF   |  25.926   46.131
D9   CK_c_A   CLK_INPUT   588.71m   1.198nH   0.562pF   |  25.948   46.170
D10   VSS   GND
D11   CA5_A   CA_INPUT   497.38m   1.012nH   0.504pF   |  22.584   44.810
D12   DQ14_A   DQ   557.46m   1.080nH   0.546pF   |  24.283   44.475
D13   VSS   GND
D14   DQS1_c_A   DQS   614.86m   1.241nH   0.581pF   |  26.852   46.217
D15   DQS1_t_A   DQS   613.28m   1.231nH   0.591pF   |  26.973   45.639
D16   VDDQ   POWER
D17   DQ8_A   DQ   485.61m   0.982nH   0.448pF   |  20.975   46.818
D18   DQ8_C   DQ   485.74m   0.981nH   0.450pF   |  21.011   46.690
D19   VDDQ   POWER
D20   DQS1_t_C   DQS   613.26m   1.233nH   0.592pF   |  27.017   45.637
D21   DQS1_c_C   DQS   616.30m   1.241nH   0.582pF   |  26.875   46.177
D22   VSS   GND
D23   DQ14_C   DQ   558.38m   1.083nH   0.547pF   |  24.339   44.496
D24   CA5_C   CA_INPUT   475.06m   0.987nH   0.484pF   |  21.857   45.158
D25   VSS   GND
D26   CK_c_C   CLK_INPUT   648.91m   1.364nH   0.609pF   |  28.821   47.326
D27   CK_t_C   CLK_INPUT   639.42m   1.334nH   0.592pF   |  28.102   47.470
D28   VSS   GND
D29   DQ6_C   DQ   564.72m   1.087nH   0.558pF   |  24.628   44.136
D30   VSS   GND
D31   DQS0_c_C   DQS   617.62m   1.252nH   0.591pF   |  27.202   46.027
D32   DQS0_t_C   DQS   619.58m   1.246nH   0.595pF   |  27.228   45.762
D33   DQ1_C   DQ   484.13m   0.949nH   0.456pF   |  20.802   45.620
D34   VDD1   POWER
E1   VDD2   POWER
E2   VSS   GND
E33   VSS   GND
E34   VDD2   POWER
F1   VDD2   POWER
F2   VDD2   POWER
F33   VDD2   POWER
F34   VDD2   POWER
G1   VSS   GND
G2   VSS   GND
G33   VSS   GND
G34   VSS   GND
H1   NC   NC
H2   NC   NC
H33   NC   NC
H34   NC   NC
J1   NC   NC
J2   NC   NC
J33   NC   NC
J34   NC   NC
K1   NC   NC
K2   NC   NC
K33   NC   NC
K34   NC   NC
L1   NC   NC
L2   NC   NC
L33   NC   NC
L34   NC   NC
M1   NC   NC
M2   NC   NC
M33   NC   NC
M34   NC   NC
N1   NC   NC
N2   NC   NC
N33   NC   NC
N34   NC   NC
P1   NC   NC
P2   NC   NC
P33   NC   NC
P34   NC   NC
R1   NC   NC
R2   NC   NC
R33   NC   NC
R34   NC   NC
T1   NC   NC
T2   NC   NC
T33   NC   NC
T34   NC   NC
U1   NC   NC
U2   NC   NC
U33   NC   NC
U34   NC   NC
V1   NC   NC
V2   NC   NC
V33   NC   NC
V34   NC   NC
W1   NC   NC
W2   NC   NC
W33   NC   NC
W34   NC   NC
Y1   NC   NC
Y2   NC   NC
Y33   NC   NC
Y34   NC   NC
AA1   NC   NC
AA2   NC   NC
AA33  NC   NC
AA34  NC   NC
AB1   NC   NC
AB2   NC   NC
AB33  NC   NC
AB34  NC   NC
AC1   NC   NC
AC2   NC   NC
AC33  NC   NC
AC34  NC   NC
AD1   NC   NC
AD2   NC   NC
AD33  NC   NC
AD34  NC   NC
AE1   NC   NC
AE2   NC   NC
AE33  NC   NC
AE34  NC   NC
AF1   NC   NC
AF2   NC   NC
AF33  NC   NC
AF34  NC   NC
AG1   NC   NC
AG2   NC   NC
AG33  NC   NC
AG34  NC   NC
AH1   VSS   GND
AH2   VSS   GND
AH33  VSS   GND
AH34  VSS   GND
AJ1   VDD2   POWER
AJ2   VDD2   POWER
AJ33  VDD2   POWER
AJ34  VDD2   POWER
AK1   VDD2   POWER
AK2   VSS   GND
AK33  VSS   GND
AK34  VDD2   POWER
AL1   VDD1   POWER
AL2   DQ1_B   DQ   500.65m   0.985nH   0.477pF   |  21.676   45.442
AL3   DQS0_t_B   DQS   635.81m   1.298nH   0.616pF   |  28.277   45.904
AL4   DQS0_c_B   DQS   634.98m   1.302nH   0.616pF   |  28.320   45.974
AL5   VSS   GND
AL6   DQ6_B   DQ   582.14m   1.132nH   0.580pF   |  25.623   44.178
AL7   VSS   GND
AL8   CK_t_B   CLK_INPUT   657.19m   1.390nH   0.614pF   |  29.214   47.580
AL9   CK_c_B   CLK_INPUT   666.55m   1.414nH   0.631pF   |  29.870   47.338
AL10  VSS   GND
AL11  CA5_B   CA_INPUT   491.81m   1.040nH   0.506pF   |  22.940   45.336
AL12  DQ14_B   DQ   575.63m   1.127nH   0.568pF   |  25.301   44.544
AL13  VSS   GND
AL14  DQS1_c_B   DQS   633.19m   1.293nH   0.604pF   |  27.946   46.268
AL15  DQS1_t_B   DQS   629.02m   1.281nH   0.613pF   |  28.022   45.713
AL16  VDDQ   POWER
AL17  DQ8_B   DQ   502.87m   1.015nH   0.472pF   |  21.888   46.373
AL18  DQ8_D   DQ   502.24m   1.017nH   0.471pF   |  21.886   46.468
AL19  VDDQ   POWER
AL20  DQS1_t_D   DQS   629.26m   1.284nH   0.612pF   |  28.032   45.804
AL21  DQS1_c_D   DQS   630.08m   1.292nH   0.603pF   |  27.912   46.288
AL22  VSS   GND
AL23  DQ14_D   DQ   574.79m   1.125nH   0.567pF   |  25.256   44.544
AL24  CA5_D   CA_INPUT   515.76m   1.066nH   0.526pF   |  23.679   45.018
AL25  VSS   GND
AL26  CK_c_D   CLK_INPUT   607.10m   1.253nH   0.584pF   |  27.051   46.320
AL27  CK_t_D   CLK_INPUT   604.00m   1.246nH   0.586pF   |  27.021   46.112
AL28  VSS   GND
AL29  DQ6_D   DQ   579.35m   1.133nH   0.579pF   |  25.613   44.236
AL30  VSS   GND
AL31  DQS0_c_D   DQS   634.81m   1.310nH   0.614pF   |  28.361   46.190
AL32  DQS0_t_D   DQS   633.54m   1.296nH   0.616pF   |  28.255   45.868
AL33  DQ1_D   DQ   498.57m   0.983nH   0.476pF   |  21.631   45.444
AL34  VDD1   POWER
AM1   DQ0_B   DQ   567.98m   1.134nH   0.526pF   |  24.423   46.432
AM2   VDDQ   POWER
AM3   VSS   GND
AM4   VSS   GND
AM5   DQ4_B   DQ   468.34m   0.914nH   0.451pF   |  20.303   45.018
AM6   VDDQ   POWER
AM7   CA1_B   CA_INPUT   437.30m   0.932nH   0.460pF   |  20.706   45.012
AM8   VDD2   POWER
AM9   VSS   GND
AM10  CA3_B   CA_INPUT   418.60m   0.906nH   0.454pF   |  20.281   44.672
AM11  VSS   GND
AM12  VDDQ   POWER
AM13  DQ12_B   DQ   452.24m   0.883nH   0.441pF   |  19.733   44.747
AM14  VSS   GND
AM15  VDDQ   POWER
AM16  DQ9_B   DQ   502.84m   0.982nH   0.479pF   |  21.688   45.278
AM17  VDD2   POWER
AM18  VDD2   POWER
AM19  DQ9_D   DQ   501.29m   0.981nH   0.479pF   |  21.677   45.255
AM20  VDDQ   POWER
AM21  VSS   GND
AM22  DQ12_D   DQ   448.71m   0.880nH   0.440pF   |  19.677   44.721
AM23  VDDQ   POWER
AM24  VSS   GND
AM25  CA3_D   CA_INPUT   445.68m   0.932nH   0.425pF   |  19.902   46.829
AM26  VSS   GND
AM27  VDD2   POWER
AM28  CA1_D   CA_INPUT   456.98m   0.971nH   0.437pF   |  20.599   47.138
AM29  VDDQ   POWER
AM30  DQ4_D   DQ   469.01m   0.918nH   0.450pF   |  20.325   45.166
AM31  VSS   GND
AM32  VSS   GND
AM33  VDDQ   POWER
AM34  DQ0_D   DQ   568.48m   1.136nH   0.527pF   |  24.468   46.428
AN1   VSS   GND
AN2   DQ2_B   DQ   563.10m   1.106nH   0.530pF   |  24.211   45.681
AN3   VDDQ   POWER
AN4   DMI0_B   DQ   541.04m   1.064nH   0.509pF   |  23.272   45.721
AN5   VDDQ   POWER
AN6   DQ7_B   DQ   521.54m   1.019nH   0.493pF   |  22.414   45.464
AN7   VDD2   POWER
AN8   CS0_B   CS_INPUT   606.77m   1.274nH   0.556pF   |  26.615   47.868
AN9   CKE0_B   CKE_INPUT   519.53m   1.095nH   0.526pF   |  23.999   45.626
AN10  VDD2   POWER
AN11  CA4_B   CA_INPUT   492.07m   1.037nH   0.522pF   |  23.266   44.571
AN12  DQ15_B   DQ   516.82m   1.002nH   0.491pF   |  22.181   45.174
AN13  VDDQ   POWER
AN14  DMI1_B   DQ   533.81m   1.053nH   0.502pF   |  22.991   45.800
AN15  DQ11_B   DQ   540.16m   1.060nH   0.509pF   |  23.228   45.635
AN16  VSS   GND
AN17  NC   NC
AN18  NC   NC
AN19  VSS   GND
AN20  DQ11_D   DQ   539.73m   1.058nH   0.509pF   |  23.206   45.592
AN21  DMI1_D   DQ   533.38m   1.056nH   0.502pF   |  23.024   45.865
AN22  VDDQ   POWER
AN23  DQ15_D   DQ   516.07m   1.015nH   0.488pF   |  22.256   45.606
AN24  CA4_D   CA_INPUT   510.48m   1.062nH   0.480pF   |  22.578   47.037
AN25  VDD2   POWER
AN26  CKE0_D   CKE_INPUT   531.26m   1.114nH   0.491pF   |  23.387   47.632
AN27  CS0_D   CS_INPUT   501.97m   1.063nH   0.471pF   |  22.376   47.507
AN28  VDD2   POWER
AN29  DQ7_D   DQ   522.87m   1.019nH   0.494pF   |  22.436   45.418
AN30  VDDQ   POWER
AN31  DMI0_D   DQ   542.52m   1.060nH   0.509pF   |  23.228   45.635
AN32  VDDQ   POWER
AN33  DQ2_D   DQ   561.84m   1.104nH   0.529pF   |  24.166   45.683
AN34  VSS   GND
AP1   NC   NC
AP2   VDD2   POWER
AP3   DQ3_B   DQ   601.27m   1.184nH   0.584pF   |  26.296   45.027
AP4   VSS   GND
AP5   DQ5_B   DQ   579.53m   1.145nH   0.567pF   |  25.480   44.938
AP6   ODT_ca_B   ODTCA_INPUT   805.14m   1.656nH   0.790pF   |  36.170   45.784
AP7   CA0_B   CA_INPUT   577.42m   1.238nH   0.607pF   |  27.413   45.161
AP10  CA2_B   CA_INPUT   576.66m   1.224nH   0.601pF   |  27.122   45.129
AP11  VSS   GND
AP12  VSS   GND
AP13  DQ13_B   DQ   587.53m   1.148nH   0.576pF   |  25.715   44.644
AP14  VDD2   POWER
AP15  VDD1   POWER
AP16  DQ10_B   DQ   611.12m   1.222nH   0.591pF   |  26.874   45.472
AP17  NC   NC
AP18  NC   NC
AP19  DQ10_D   DQ   610.56m   1.226nH   0.589pF   |  26.872   45.623
AP20  VDD1   POWER
AP21  VDD2   POWER
AP22  DQ13_D   DQ   586.50m   1.152nH   0.575pF   |  25.737   44.760
AP23  VSS   GND
AP24  VSS   GND
AP25  CA2_D   CA_INPUT   569.00m   1.202nH   0.550pF   |  25.712   46.749
AP28  CA0_D   CA_INPUT   604.13m   1.274nH   0.576pF   |  27.089   47.030
AP29  ODT_ca_D   ODTCA_INPUT   605.04m   1.258nH   0.572pF   |  26.825   46.897
AP30  DQ5_D   DQ   580.85m   1.145nH   0.567pF   |  25.480   44.938
AP31  VSS   GND
AP32  DQ3_D   DQ   599.52m   1.181nH   0.583pF   |  26.240   45.008
AP33  VDD2   POWER
AP34  NC   NC
|*****  PIN MAPPING  *******************************************************
[Pin Mapping] pulldown_ref pullup_ref gnd_clamp_ref power_clamp_ref ext_ref
A1   NC   NC
A2   NC   VDD2
A3   VSS   VDDQ   VSS   VDDQ
A4   VSS   NC
A5   VSS   VDDQ   VSS   VDDQ
A6   NC   NC   VSS   VDD2
A7   NC   NC   VSS   VDD2
A10   NC   NC   VSS   VDD2
A11   VSS   NC
A12   VSS   NC
A13   VSS   VDDQ   VSS   VDDQ
A14   NC   VDD2
A15   NC   VDD1
A16   VSS   VDDQ   VSS   VDDQ
A17   NC   NC
A18   NC   NC
A19   VSS   VDDQ   VSS   VDDQ
A20   NC   VDD1
A21   NC   VDD2
A22   VSS   VDDQ   VSS   VDDQ
A23   VSS   NC
A24   VSS   NC
A25   NC   NC   VSS   VDD2
A28   NC   NC   VSS   VDD2
A29   NC   NC   VSS   VDD2
A30   VSS   VDDQ   VSS   VDDQ
A31   VSS   NC
A32   VSS   VDDQ   VSS   VDDQ
A33   NC   VDD2
A34   NC   NC
B1   VSS   NC
B2   VSS   VDDQ   VSS   VDDQ
B3   NC   VDDQ
B4   VSS   VDDQ   VSS   VDDQ
B5   NC   VDDQ
B6   VSS   VDDQ   VSS   VDDQ
B7   NC   VDD2
B8   NC   NC   VSS   VDD2
B9   NC   NC   VSS   VDD2
B10   NC   VDD2
B11   NC   NC   VSS   VDD2
B12   VSS   VDDQ   VSS   VDDQ
B13   NC   VDDQ
B14   VSS   VDDQ   VSS   VDDQ
B15   VSS   VDDQ   VSS   VDDQ
B16   VSS   NC
B17   NC   NC
B18   NC   NC
B19   VSS   NC
B20   VSS   VDDQ   VSS   VDDQ
B21   VSS   VDDQ   VSS   VDDQ
B22   NC   VDDQ
B23   VSS   VDDQ   VSS   VDDQ
B24   NC   NC   VSS   VDD2
B25   NC   VDD2
B26   NC   NC   VSS   VDD2
B27   NC   NC   VSS   VDD2
B28   NC   VDD2
B29   VSS   VDDQ   VSS   VDDQ
B30   NC   VDDQ
B31   VSS   VDDQ   VSS   VDDQ
B32   NC   VDDQ
B33   VSS   VDDQ   VSS   VDDQ
B34   VSS   NC
C1   VSS   VDDQ   VSS   VDDQ
C2   NC   VDDQ
C3   VSS   NC
C4   VSS   NC
C5   VSS   VDDQ   VSS   VDDQ
C6   NC   VDDQ
C7   NC   NC   VSS   VDD2
C8   NC   VDD2
C9   VSS   NC
C10   NC   NC   VSS   VDD2
C11   VSS   NC
C12   NC   VDDQ
C13   VSS   VDDQ   VSS   VDDQ
C14   VSS   NC
C15   NC   VDDQ
C16   VSS   VDDQ   VSS   VDDQ
C17   NC   NC
C18   NC   NC
C19   VSS   VDDQ   VSS   VDDQ
C20   NC   VDDQ
C21   VSS   NC
C22   VSS   VDDQ   VSS   VDDQ
C23   NC   VDDQ
C24   VSS   NC
C25   NC   NC   VSS   VDD2
C26   VSS   NC
C27   NC   VDD2
C28   NC   NC   VSS   VDD2
C29   NC   VDDQ
C30   VSS   VDDQ   VSS   VDDQ
C31   VSS   NC
C32   VSS   NC
C33   NC   VDDQ
C34   VSS   VDDQ   VSS   VDDQ
D1   NC   VDD1
D2   VSS   VDDQ   VSS   VDDQ
D3   VSS   VDDQ   VSS   VDDQ
D4   VSS   VDDQ   VSS   VDDQ
D5   VSS   NC
D6   VSS   VDDQ   VSS   VDDQ
D7   VSS   NC
D8   NC   NC   VSS   VDD2
D9   NC   NC   VSS   VDD2
D10   VSS   NC
D11   NC   NC   VSS   VDD2
D12   VSS   VDDQ   VSS   VDDQ
D13   VSS   NC
D14   VSS   VDDQ   VSS   VDDQ
D15   VSS   VDDQ   VSS   VDDQ
D16   NC   VDDQ
D17   VSS   VDDQ   VSS   VDDQ
D18   VSS   VDDQ   VSS   VDDQ
D19   NC   VDDQ
D20   VSS   VDDQ   VSS   VDDQ
D21   VSS   VDDQ   VSS   VDDQ
D22   VSS   NC
D23   VSS   VDDQ   VSS   VDDQ
D24   NC   NC   VSS   VDD2
D25   VSS   NC
D26   NC   NC   VSS   VDD2
D27   NC   NC   VSS   VDD2
D28   VSS   NC
D29   VSS   VDDQ   VSS   VDDQ
D30   VSS   NC
D31   VSS   VDDQ   VSS   VDDQ
D32   VSS   VDDQ   VSS   VDDQ
D33   VSS   VDDQ   VSS   VDDQ
D34   NC   VDD1
E1   NC   VDD2
E2   VSS   NC
E33   VSS   NC
E34   NC   VDD2
F1   NC   VDD2
F2   NC   VDD2
F33   NC   VDD2
F34   NC   VDD2
G1   VSS   NC
G2   VSS   NC
G33   VSS   NC
G34   VSS   NC
H1   NC   NC
H2   NC   NC
H33   NC   NC
H34   NC   NC
J1   NC   NC
J2   NC   NC
J33   NC   NC
J34   NC   NC
K1   NC   NC
K2   NC   NC
K33   NC   NC
K34   NC   NC
L1   NC   NC
L2   NC   NC
L33   NC   NC
L34   NC   NC
M1   NC   NC
M2   NC   NC
M33   NC   NC
M34   NC   NC
N1   NC   NC
N2   NC   NC
N33   NC   NC
N34   NC   NC
P1   NC   NC
P2   NC   NC
P33   NC   NC
P34   NC   NC
R1   NC   NC
R2   NC   NC
R33   NC   NC
R34   NC   NC
T1   NC   NC
T2   NC   NC
T33   NC   NC
T34   NC   NC
U1   NC   NC
U2   NC   NC
U33   NC   NC
U34   NC   NC
V1   NC   NC
V2   NC   NC
V33   NC   NC
V34   NC   NC
W1   NC   NC
W2   NC   NC
W33   NC   NC
W34   NC   NC
Y1   NC   NC
Y2   NC   NC
Y33   NC   NC
Y34   NC   NC
AA1   NC   NC
AA2   NC   NC
AA33   NC   NC
AA34   NC   NC
AB1   NC   NC
AB2   NC   NC
AB33   NC   NC
AB34   NC   NC
AC1   NC   NC
AC2   NC   NC
AC33   NC   NC
AC34   NC   NC
AD1   NC   NC
AD2   NC   NC
AD33   NC   NC
AD34   NC   NC
AE1   NC   NC
AE2   NC   NC
AE33   NC   NC
AE34   NC   NC
AF1   NC   NC
AF2   NC   NC
AF33   NC   NC
AF34   NC   NC
AG1   NC   NC
AG2   NC   NC
AG33   NC   NC
AG34   NC   NC
AH1   VSS   NC
AH2   VSS   NC
AH33   VSS   NC
AH34   VSS   NC
AJ1   NC   VDD2
AJ2   NC   VDD2
AJ33   NC   VDD2
AJ34   NC   VDD2
AK1   NC   VDD2
AK2   VSS   NC
AK33   VSS   NC
AK34   NC   VDD2
AL1   NC   VDD1
AL2   VSS   VDDQ   VSS   VDDQ
AL3   VSS   VDDQ   VSS   VDDQ
AL4   VSS   VDDQ   VSS   VDDQ
AL5   VSS   NC
AL6   VSS   VDDQ   VSS   VDDQ
AL7   VSS   NC
AL8   NC   NC   VSS   VDD2
AL9   NC   NC   VSS   VDD2
AL10   VSS   NC
AL11   NC   NC   VSS   VDD2
AL12   VSS   VDDQ   VSS   VDDQ
AL13   VSS   NC
AL14   VSS   VDDQ   VSS   VDDQ
AL15   VSS   VDDQ   VSS   VDDQ
AL16   NC   VDDQ
AL17   VSS   VDDQ   VSS   VDDQ
AL18   VSS   VDDQ   VSS   VDDQ
AL19   NC   VDDQ
AL20   VSS   VDDQ   VSS   VDDQ
AL21   VSS   VDDQ   VSS   VDDQ
AL22   VSS   NC
AL23   VSS   VDDQ   VSS   VDDQ
AL24   NC   NC   VSS   VDD2
AL25   VSS   NC
AL26   NC   NC   VSS   VDD2
AL27   NC   NC   VSS   VDD2
AL28   VSS   NC
AL29   VSS   VDDQ   VSS   VDDQ
AL30   VSS   NC
AL31   VSS   VDDQ   VSS   VDDQ
AL32   VSS   VDDQ   VSS   VDDQ
AL33   VSS   VDDQ   VSS   VDDQ
AL34   NC   VDD1
AM1   VSS   VDDQ   VSS   VDDQ
AM2   NC   VDDQ
AM3   VSS   NC
AM4   VSS   NC
AM5   VSS   VDDQ   VSS   VDDQ
AM6   NC   VDDQ
AM7   NC   NC   VSS   VDD2
AM8   NC   VDD2
AM9   VSS   NC
AM10   NC   NC   VSS   VDD2
AM11   VSS   NC
AM12   NC   VDDQ
AM13   VSS   VDDQ   VSS   VDDQ
AM14   VSS   NC
AM15   NC   VDDQ
AM16   VSS   VDDQ   VSS   VDDQ
AM17   NC   VDD2
AM18   NC   VDD2
AM19   VSS   VDDQ   VSS   VDDQ
AM20   NC   VDDQ
AM21   VSS   NC
AM22   VSS   VDDQ   VSS   VDDQ
AM23   NC   VDDQ
AM24   VSS   NC
AM25   NC   NC   VSS   VDD2
AM26   VSS   NC
AM27   NC   VDD2
AM28   NC   NC   VSS   VDD2
AM29   NC   VDDQ
AM30   VSS   VDDQ   VSS   VDDQ
AM31   VSS   NC
AM32   VSS   NC
AM33   NC   VDDQ
AM34   VSS   VDDQ   VSS   VDDQ
AN1   VSS   NC
AN2   VSS   VDDQ   VSS   VDDQ
AN3   NC   VDDQ
AN4   VSS   VDDQ   VSS   VDDQ
AN5   NC   VDDQ
AN6   VSS   VDDQ   VSS   VDDQ
AN7   NC   VDD2
AN8   NC   NC   VSS   VDD2
AN9   NC   NC   VSS   VDD2
AN10   NC   VDD2
AN11   NC   NC   VSS   VDD2
AN12   VSS   VDDQ   VSS   VDDQ
AN13   NC   VDDQ
AN14   VSS   VDDQ   VSS   VDDQ
AN15   VSS   VDDQ   VSS   VDDQ
AN16   VSS   NC
AN17   NC   NC
AN18   NC   NC
AN19   VSS   NC
AN20   VSS   VDDQ   VSS   VDDQ
AN21   VSS   VDDQ   VSS   VDDQ
AN22   NC   VDDQ
AN23   VSS   VDDQ   VSS   VDDQ
AN24   NC   NC   VSS   VDD2
AN25   NC   VDD2
AN26   NC   NC   VSS   VDD2
AN27   NC   NC   VSS   VDD2
AN28   NC   VDD2
AN29   VSS   VDDQ   VSS   VDDQ
AN30   NC   VDDQ
AN31   VSS   VDDQ   VSS   VDDQ
AN32   NC   VDDQ
AN33   VSS   VDDQ   VSS   VDDQ
AN34   VSS   NC
AP1   NC   NC
AP2   NC   VDD2
AP3   VSS   VDDQ   VSS   VDDQ
AP4   VSS   NC
AP5   VSS   VDDQ   VSS   VDDQ
AP6   NC   NC   VSS   VDD2
AP7   NC   NC   VSS   VDD2
AP10   NC   NC   VSS   VDD2
AP11   VSS   NC
AP12   VSS   NC
AP13   VSS   VDDQ   VSS   VDDQ
AP14   NC   VDD2
AP15   NC   VDD1
AP16   VSS   VDDQ   VSS   VDDQ
AP17   NC   NC
AP18   NC   NC
AP19   VSS   VDDQ   VSS   VDDQ
AP20   NC   VDD1
AP21   NC   VDD2
AP22   VSS   VDDQ   VSS   VDDQ
AP23   VSS   NC
AP24   VSS   NC
AP25   NC   NC   VSS   VDD2
AP28   NC   NC   VSS   VDD2
AP29   NC   NC   VSS   VDD2
AP30   VSS   VDDQ   VSS   VDDQ
AP31   VSS   NC
AP32   VSS   VDDQ   VSS   VDDQ
AP33   NC   VDD2
AP34   NC   NC
|*****  DIFF PIN  **********************************************************
[Diff Pin]  inv_pin  vdiff   tdelay_typ   tdelay_min   tdelay_max
D3   D4   0.120V   0.000s   NA   NA
D32   D31   0.120V   0.000s   NA   NA
AL3   AL4   0.120V   0.000s   NA   NA
AL32   AL31   0.120V   0.000s   NA   NA
D15   D14   0.120V   0.000s   NA   NA
D20   D21   0.120V   0.000s   NA   NA
AL15   AL14   0.120V   0.000s   NA   NA
AL20   AL21   0.120V   0.000s   NA   NA
D8   D9   0.145V   0.000s   NA   NA
D27   D26   0.145V   0.000s   NA   NA
AL8   AL9   0.145V   0.000s   NA   NA
AL27   AL26   0.145V   0.000s   NA   NA
|END COMPONENT *************************************************************
|COMPONENT:[ MT53E1G64D4NW ]
[Component]   MT53E1G64D4NW
[Package Model]  Z42N_432B_PKG
[Manufacturer]   xxx Technology, Inc.
[Package]
|   typ   min   max
R_pkg   497.93m   363.79m   923.96m
L_pkg   1.024nH   0.757nH   1.955nH
C_pkg   0.449pF   0.326pF   0.792pF
[Pin] signal_name  model_name   R_pin   L_pin   C_pin   | TD_pin(ps)   Z_pin
A1   VDDQ   POWER
A2   VDD1   POWER
A3   VDDQ   POWER
A4   VDDQ   POWER
A5   VDDQ   POWER
A6   VDD2   POWER
A8   VDD2   POWER
A9   VDDQ   POWER
A10   VDDQ   POWER
A11   VDDQ   POWER
A12   VDD1   POWER
A13   VDDQ   POWER
A15   VDDQ   POWER
A16   VDD1   POWER
A17   VDDQ   POWER
A18   VDDQ   POWER
A19   VDDQ   POWER
A20   VDD2   POWER
A22   VDD2   POWER
A23   VDDQ   POWER
A24   VDDQ   POWER
A25   VDDQ   POWER
A26   VDD1   POWER
A27   VDDQ   POWER
B1   VDDQ   POWER
B2   VDD1   POWER
B3   DQ0_A   DQ   393.64m   0.787nH   0.346pF   |  16.502   47.692
B4   VSS   GND
B5   CA0_A   CA_INPUT   447.07m   0.962nH   0.432pF   |  20.386   47.190
B6   VDD2   POWER
B8   VDD2   POWER
B9   CA4_A   CA_INPUT   419.09m   0.910nH   0.407pF   |  19.245   47.285
B10   VSS   GND
B11   DQ8_A   DQ   374.23m   0.757nH   0.326pF   |  15.709   48.188
B12   VDD1   POWER
B13   VDDQ   POWER
B15   VDDQ   POWER
B16   VDD1   POWER
B17   DQ0_C   DQ   393.82m   0.787nH   0.346pF   |  16.502   47.692
B18   VSS   GND
B19   CA0_C   CA_INPUT   447.25m   0.967nH   0.426pF   |  20.296   47.644
B20   VDD2   POWER
B22   VDD2   POWER
B23   CA4_C   CA_INPUT   419.26m   0.910nH   0.408pF   |  19.269   47.227
B24   VSS   GND
B25   DQ8_C   DQ   374.41m   0.758nH   0.326pF   |  15.720   48.220
B26   VDD1   POWER
B27   VDDQ   POWER
C1   VDDQ   POWER
C2   DQ1_A   DQ   397.13m   0.789nH   0.390pF   |  17.542   44.979
C3   VSS   GND
C4   DQ5_A   DQ   498.67m   0.991nH   0.477pF   |  21.742   45.580
C5   VSS   GND
C6   CA2_A   CA_INPUT   427.31m   0.921nH   0.419pF   |  19.644   46.884
C8   CA3_A   CA_INPUT   368.51m   0.781nH   0.375pF   |  17.114   45.636
C9   VSS   GND
C10   DQ13_A   DQ   509.73m   1.032nH   0.479pF   |  22.233   46.416
C11   VSS   GND
C12   DQ9_A   DQ   379.38m   0.772nH   0.381pF   |  17.150   45.014
C13   VDDQ   POWER
C15   VDDQ   POWER
C16   DQ1_C   DQ   397.31m   0.790nH   0.393pF   |  17.620   44.835
C17   VSS   GND
C18   DQ5_C   DQ   498.85m   0.993nH   0.477pF   |  21.764   45.626
C19   VSS   GND
C20   CA2_C   CA_INPUT   427.48m   0.921nH   0.416pF   |  19.574   47.053
C22   CA3_C   CA_INPUT   368.68m   0.781nH   0.375pF   |  17.114   45.636
C23   VSS   GND
C24   DQ13_C   DQ   509.91m   1.032nH   0.479pF   |  22.233   46.416
C25   VSS   GND
C26   DQ9_C   DQ   379.55m   0.773nH   0.382pF   |  17.184   44.984
C27   VDDQ   POWER
D1   VDDQ   POWER
D2   VSS   GND
D3   DQ4_A   DQ   543.18m   1.077nH   0.519pF   |  23.642   45.554
D4   VSS   GND
D5   CA1_A   CA_INPUT   516.08m   1.088nH   0.497pF   |  23.254   46.788
D6   VDD2   POWER
D8   VDD2   POWER
D9   CA5_A   CA_INPUT   475.48m   1.008nH   0.465pF   |  21.650   46.559
D10   VSS   GND
D11   DQ12_A   DQ   573.51m   1.151nH   0.537pF   |  24.861   46.297
D12   VSS   GND
D13   VDDQ   POWER
D15   VDDQ   POWER
D16   VSS   GND
D17   DQ4_C   DQ   543.34m   1.078nH   0.519pF   |  23.653   45.575
D18   VSS   GND
D19   CA1_C   CA_INPUT   512.35m   1.088nH   0.497pF   |  23.254   46.788
D20   VDD2   POWER
D22   VDD2   POWER
D23   CA5_C   CA_INPUT   475.66m   1.008nH   0.464pF   |  21.627   46.609
D24   VSS   GND
D25   DQ12_C   DQ   573.68m   1.151nH   0.538pF   |  24.884   46.254
D26   VSS   GND
D27   VDDQ   POWER
E1   VDDQ   POWER
E2   DQ2_A   DQ   440.39m   0.841nH   0.378pF   |  17.830   47.169
E3   VSS   GND
E4   DQ6_A   DQ   406.69m   0.793nH   0.405pF   |  17.921   44.250
E5   VSS   GND
E6   CK_t_A   CLK_INPUT   368.48m   0.759nH   0.380pF   |  16.983   44.692
E8   CK_c_A   CLK_INPUT   386.00m   0.788nH   0.374pF   |  17.167   45.902
E9   VSS   GND
E10   DQ14_A   DQ   424.34m   0.830nH   0.417pF   |  18.604   44.614
E11   VSS   GND
E12   DQ10_A   DQ   439.92m   0.862nH   0.375pF   |  17.979   47.944
E13   VDDQ   POWER
E15   VDDQ   POWER
E16   DQ2_C   DQ   440.54m   0.842nH   0.378pF   |  17.840   47.197
E17   VSS   GND
E18   DQ6_C   DQ   406.86m   0.792nH   0.405pF   |  17.910   44.222
E19   VSS   GND
E20   CK_t_C   CLK_INPUT   363.79m   0.760nH   0.382pF   |  17.039   44.604
E22   CK_c_C   CLK_INPUT   376.91m   0.785nH   0.374pF   |  17.134   45.814
E23   VSS   GND
E24   DQ14_C   DQ   424.51m   0.831nH   0.417pF   |  18.615   44.641
E25   VSS   GND
E26   DQ10_C   DQ   440.09m   0.862nH   0.375pF   |  17.979   47.944
E27   VDDQ   POWER
F1   VDDQ   POWER
F2   VSS   GND
F3   DQS0_t_A   DQS   496.38m   1.039nH   0.460pF   |  21.862   47.526
F4   VSS   GND
F5   NC   NC
F6   VDD2   POWER
F8   VDD2   POWER
F9   CKE0_A   CKE_INPUT   604.26m   1.307nH   0.552pF   |  26.860   48.660
F10   VSS   GND
F11   DQS1_t_A   DQS   485.19m   1.024nH   0.460pF   |  21.703   47.181
F12   VSS   GND
F13   VDDQ   POWER
F15   VDDQ   POWER
F16   VSS   GND
F17   DQS0_t_C   DQS   496.57m   1.040nH   0.460pF   |  21.872   47.549
F18   VSS   GND
F19   NC   NC
F20   VDD2   POWER
F22   VDD2   POWER
F23   CKE0_C   CKE_INPUT   604.43m   1.308nH   0.552pF   |  26.870   48.678
F24   VSS   GND
F25   DQS1_t_C   DQS   485.32m   1.028nH   0.459pF   |  21.722   47.325
F26   VSS   GND
F27   VDDQ   POWER
G1   VDDQ   POWER
G2   DQ3_A   DQ   541.67m   1.070nH   0.445pF   |  21.821   49.036
G3   VSS   GND
G4   DQS0_c_A   DQS   489.60m   1.005nH   0.452pF   |  21.313   47.153
G5   VSS   GND
G6   CS0_A   CS_INPUT   486.51m   1.030nH   0.414pF   |  20.650   49.879
G8   NC   NC
G9   VSS   GND
G10   DQS1_c_A   DQS   484.27m   1.005nH   0.445pF   |  21.148   47.523
G11   VSS   GND
G12   DQ11_A   DQ   556.19m   1.109nH   0.455pF   |  22.463   49.370
G13   VDDQ   POWER
G15   VDDQ   POWER
G16   DQ3_C   DQ   541.84m   1.072nH   0.444pF   |  21.817   49.137
G17   VSS   GND
G18   DQS0_c_C   DQS   489.79m   1.008nH   0.450pF   |  21.298   47.329
G19   VSS   GND
G20   CS0_C   CS_INPUT   486.69m   1.030nH   0.414pF   |  20.650   49.879
G22   NC   NC
G23   VSS   GND
G24   DQS1_c_C   DQS   484.38m   1.007nH   0.448pF   |  21.240   47.411
G25   VSS   GND
G26   DQ11_C   DQ   556.36m   1.112nH   0.454pF   |  22.469   49.491
G27   VDDQ   POWER
H1   VDDQ   POWER
H2   VSS   GND
H3   DMI0_A   DQ   622.39m   1.230nH   0.507pF   |  24.972   49.255
H4   VSS   GND
H5   DQ7_A   DQ   569.15m   1.124nH   0.469pF   |  22.960   48.955
H6   VDD2   POWER
H8   VDD2   POWER
H9   DQ15_A   DQ   577.15m   1.162nH   0.468pF   |  23.320   49.829
H10   VSS   GND
H11   DMI1_A   DQ   615.97m   1.237nH   0.499pF   |  24.845   49.789
H12   VSS   GND
H13   VDDQ   POWER
H15   VDDQ   POWER
H16   VSS   GND
H17   DMI0_C   DQ   622.54m   1.231nH   0.507pF   |  24.982   49.275
H18   VSS   GND
H19   DQ7_C   DQ   569.30m   1.129nH   0.469pF   |  23.011   49.064
H20   VDD2   POWER
H22   VDD2   POWER
H23   DQ15_C   DQ   577.40m   1.165nH   0.469pF   |  23.375   49.840
H24   VSS   GND
H25   DMI1_C   DQ   616.18m   1.221nH   0.504pF   |  24.807   49.220
H26   VSS   GND
H27   VDDQ   POWER
J1   VDDQ   POWER
J2   NC   NC
J3   NC   NC
J4   ODT_CA_A   ODTCA_INPUT   763.66m   1.618nH   0.661pF   |  32.703   49.475
J5   NC   NC
J6   NC   NC
J8   NC   NC
J9   NC   NC
J10   ZQ0_A   NC
J11   VSS   GND
J12   NC   NC
J13   VDDQ   POWER
J15   VDDQ   POWER
J16   NC   NC
J17   NC   NC
J18   ODT_CA_C   ODTCA_INPUT   763.81m   1.623nH   0.654pF   |  32.580   49.816
J19   NC   NC
J20   NC   NC
J22   NC   NC
J23   NC   NC
J24   ZQ0_C   NC
J25   VSS   GND
J26   NC   NC
J27   VDDQ   POWER
U1   VDDQ   POWER
U2   VSS   GND
U3   VSS   GND
U4   ODT_CA_B   ODTCA_INPUT   923.82m   1.948nH   0.792pF   |  39.279   49.594
U5   NC   NC
U6   NC   NC
U8   NC   NC
U9   NC   NC
U10   VSS   GND
U11   VSS   GND
U12   RESET_n   NC
U13   VDDQ   POWER
U15   VDDQ   POWER
U16   VSS   GND
U17   VSS   GND
U18   ODT_CA_D   ODTCA_INPUT   923.96m   1.955nH   0.789pF   |  39.275   49.778
U19   NC   NC
U20   NC   NC
U22   NC   NC
U23   NC   NC
U24   VSS   GND
U25   VSS   GND
U26   NC   NC
U27   VDDQ   POWER
V1   VDDQ   POWER
V2   VSS   GND
V3   DMI0_B   DQ   627.97m   1.270nH   0.506pF   |  25.350   50.099
V4   VSS   GND
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| Models and submodels in the file (175): DQ_PD40_SOC-ODT40_VOH30_4266 (I/O), DQ_PD40_SOC-ODT48_VOH30_4266 (I/O), DQ_PD40_SOC-ODT60_VOH30_4266 (I/O), DQ_PD40_SOC-ODT80_VOH30_4266 (I/O), DQ_PD40_SOC-ODT120_VOH30_4266 (I/O), DQ_PD40_SOC-ODT240_VOH30_4266 (I/O), DQ_PD40_SOC-ODTDIS_VOH30_4266 (I/O), DQ_PD40_SOC-ODT80_VOH25_4266 (I/O), DQ_PD40_SOC-ODT120_VOH25_4266 (I/O), DQ_PD40_SOC-ODT240_VOH25_4266 (I/O), DQ_PD40_SOC-ODTDIS_VOH25_4266 (I/O), DQ_PD48_SOC-ODT40_VOH30_4266 (I/O), DQ_PD48_SOC-ODT48_VOH30_4266 (I/O), DQ_PD48_SOC-ODT60_VOH30_4266 (I/O), DQ_PD48_SOC-ODT80_VOH30_4266 (I/O), DQ_PD48_SOC-ODT120_VOH30_4266 (I/O), DQ_PD48_SOC-ODT240_VOH30_4266 (I/O), DQ_PD48_SOC-ODTDIS_VOH30_4266 (I/O), DQ_PD48_SOC-ODT80_VOH25_4266 (I/O), DQ_PD48_SOC-ODT120_VOH25_4266 (I/O), DQ_PD48_SOC-ODT240_VOH25_4266 (I/O), DQ_PD48_SOC-ODTDIS_VOH25_4266 (I/O), DQ_PD60_SOC-ODT40_VOH30_4266 (I/O), DQ_PD60_SOC-ODT48_VOH30_4266 (I/O), DQ_PD60_SOC-ODT60_VOH30_4266 (I/O), DQ_PD60_SOC-ODT80_VOH30_4266 (I/O), DQ_PD60_SOC-ODT120_VOH30_4266 (I/O), DQ_PD60_SOC-ODT240_VOH30_4266 (I/O), DQ_PD60_SOC-ODTDIS_VOH30_4266 (I/O), DQ_PD60_SOC-ODT80_VOH25_4266 (I/O), DQ_PD60_SOC-ODT120_VOH25_4266 (I/O), DQ_PD60_SOC-ODT240_VOH25_4266 (I/O), DQ_PD60_SOC-ODTDIS_VOH25_4266 (I/O), DQ_PD80_SOC-ODT40_VOH30_4266 (I/O), DQ_PD80_SOC-ODT48_VOH30_4266 (I/O), DQ_PD80_SOC-ODT60_VOH30_4266 (I/O), DQ_PD80_SOC-ODT80_VOH30_4266 (I/O), DQ_PD80_SOC-ODT120_VOH30_4266 (I/O), DQ_PD80_SOC-ODT240_VOH30_4266 (I/O), DQ_PD80_SOC-ODTDIS_VOH30_4266 (I/O), DQ_PD80_SOC-ODT80_VOH25_4266 (I/O), DQ_PD80_SOC-ODT120_VOH25_4266 (I/O), DQ_PD80_SOC-ODT240_VOH25_4266 (I/O), DQ_PD80_SOC-ODTDIS_VOH25_4266 (I/O), DQ_PD120_SOC-ODT40_VOH30_4266 (I/O), DQ_PD120_SOC-ODT48_VOH30_4266 (I/O), DQ_PD120_SOC-ODT60_VOH30_4266 (I/O), DQ_PD120_SOC-ODT80_VOH30_4266 (I/O), DQ_PD120_SOC-ODT120_VOH30_4266 (I/O), DQ_PD120_SOC-ODT240_VOH30_4266 (I/O), DQ_PD120_SOC-ODTDIS_VOH30_4266 (I/O), DQ_PD120_SOC-ODT80_VOH25_4266 (I/O), DQ_PD120_SOC-ODT120_VOH25_4266 (I/O), DQ_PD120_SOC-ODT240_VOH25_4266 (I/O), DQ_PD120_SOC-ODTDIS_VOH25_4266 (I/O), DQ_PD240_SOC-ODT40_VOH30_4266 (I/O), DQ_PD240_SOC-ODT48_VOH30_4266 (I/O), DQ_PD240_SOC-ODT60_VOH30_4266 (I/O), DQ_PD240_SOC-ODT80_VOH30_4266 (I/O), DQ_PD240_SOC-ODT120_VOH30_4266 (I/O), DQ_PD240_SOC-ODT240_VOH30_4266 (I/O), DQ_PD240_SOC-ODTDIS_VOH30_4266 (I/O), DQ_PD240_SOC-ODT80_VOH25_4266 (I/O), DQ_PD240_SOC-ODT120_VOH25_4266 (I/O), DQ_PD240_SOC-ODT240_VOH25_4266 (I/O), DQ_PD240_SOC-ODTDIS_VOH25_4266 (I/O), DQ_IN_ODTOFF_4266 (Input), DQ_IN_ODT40_4266 (Input), DQ_IN_ODT48_4266 (Input), DQ_IN_ODT60_4266 (Input), DQ_IN_ODT80_4266 (Input), DQ_IN_ODT120_4266 (Input), DQ_IN_ODT240_4266 (Input), DQS_PD40_SOC-ODT40_VOH30_4266 (I/O), DQS_PD40_SOC-ODT48_VOH30_4266 (I/O), DQS_PD40_SOC-ODT60_VOH30_4266 (I/O), DQS_PD40_SOC-ODT80_VOH30_4266 (I/O), DQS_PD40_SOC-ODT120_VOH30_4266 (I/O), DQS_PD40_SOC-ODT240_VOH30_4266 (I/O), DQS_PD40_SOC-ODTDIS_VOH30_4266 (I/O)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
